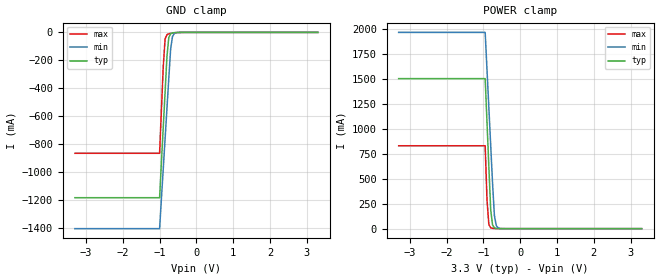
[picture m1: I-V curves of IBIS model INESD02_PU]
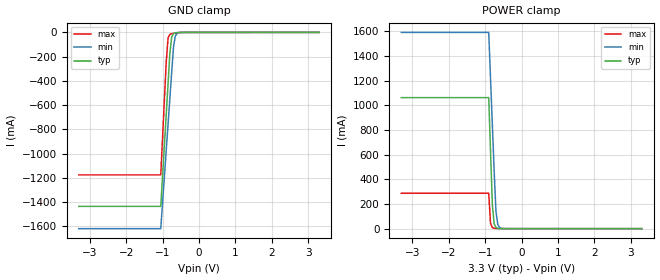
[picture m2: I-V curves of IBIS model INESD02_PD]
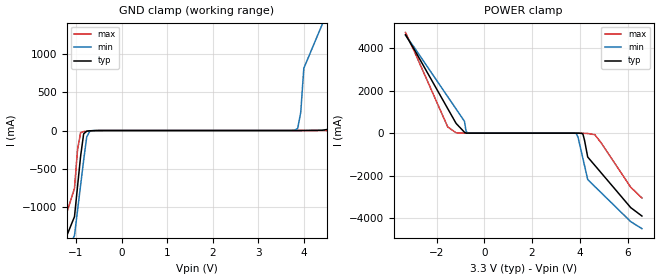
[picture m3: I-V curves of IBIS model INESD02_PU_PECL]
|   This file is an IBIS representation of the   |
|   Integrated Device Technology, Inc.   |
|   ICS844003EI-01   |
|   FEMTOCLOCKS CRYSTAL-TO-LVDS FREQUENCY SYNTHESIZER   |
[IBIS Ver]   4.1
[File name]   844003ei_01_3v3.ibs
[File Rev]   1.0
[Date]   20 Aug 2010
[Source]   Originated at Integrated Device Technology, Inc.
[Disclaimer]
IDT hereby grants the user of this IBIS model a non-exclusive,
nontransferable license to use this IBIS model under the following terms.
Before using this IBIS model, the user should read this license.
If the user does not accept these terms,  the IBIS model should be
returned to IDT within 30 days.
   The user is granted this license only to use the IBIS model and
is not granted rights to sell, load, rent, lease or license the IBIS
model in whole or in part, or in modified form to anyone other than
user. User may modify the IBIS model to suit its specific
applications but rights to derivative works and such modifications
shall belong to IDT.
   This IBIS model is provided on an "AS IS" basis and IDT makes
absolutely no warranty with respect to the information contained
herein. IDT DISCLAIMS AND CUSTOMER WAIVES ALL WARRANTIES, EXPRESS
OR IMPLIED, INCLUDING WARRANTIES OF MERCHANTABILITY OR FITNESS FOR
A PARTICULAR PURPOSE. The entire risk as to quality and performance
is with the Customer. ACCORDINGLY, IN NO EVENT SHALL THE COMPANY BE
LIABLE FOR ANY DAMAGES, WHETHER IN CONTRACT OR TORT,INCLUDING ANY
LOST PROFITS OR OTHER INCIDENTAL, CONSEQUENTIAL, EXEMPLARY, OR
PUNITIVE DAMAGES ARISING OUT OF THE USE OR APPLICATION OF THE IBIS
model provided in this package. Further, IDT reserves the right to
make changes without notice to any product herein to improve
reliability, function, or design. IDT does not convey any license
under patent rights or any other intellectual property rights,
including those of third parties.
   IDT is not obligated to provide maintenance or support
for the licensed IBIS model.
[Copyright]   Copyright 2010 by Integrated Device Technology, Inc.
[Component]   ICS844003EGI-01
[Manufacturer] Integrated Device Technology, Inc.
[Package]
|TSSOP 24 Lead
|   typ   min   max
R_pkg   60.65m   52.4m   68.9m
L_pkg   1.989nH   1.431nH   2.547nH
C_pkg   0.314pF   0.254pF   0.374pF
[Pin] signal_name  model_name   R_pin   L_pin   C_pin
1   DIV_SEL0   INESD02_PU   68.9m   2.547n   0.374p
2   VCO_SEL   INESD02_PU   65.6m   2.323n   0.350p
3   MR   INESD02_PD   62.3m   2.100n   0.326p
4   NC   NC   59.0m   1.877n   0.302p
5   NC   NC   55.7m   1.654n   0.278p
6   NC   NC   52.4m   1.431n   0.254p
7   OE   INESD02_PU_PECL   52.4m   1.431n   0.254p
8   NC   NC   55.7m   1.654n   0.278p
9   FB_DIV   INESD02_PD   59.0m   1.877n   0.302p
10   VDDA   POWER   62.3m   2.100n   0.326p
11   VDD   POWER   65.6m   2.323n   0.350p
12   NC   NC   68.9m   2.547n   0.374p
13   NC   NC   68.9m   2.547n   0.374p
14   GND   GND   65.6m   2.323n   0.350p
15   XTAL_OUT   NC   62.3m   2.100n   0.326p
16   XTAL_IN   NC   59.0m   1.877n   0.302p
17   REF_CLK   INESD02_PD_PECL   55.7m   1.654n   0.278p
18   XTAL_SEL   INESD02_PU   52.4m   1.431n   0.254p
19   nQ1   ONLVDS03_LVDS01_   52.4m   1.431n   0.254p
20   Q1   ONLVDS03_LVDS01_   55.7m   1.654n   0.278p
21   nQ0   ONLVDS03_LVDS01_   59.0m   1.877n   0.302p
22   Q0   ONLVDS03_LVDS01_   62.3m   2.100n   0.326p
23   VDDO   POWER   65.6m   2.323n   0.350p
24   DIV_SEL1   INESD02_PU   68.9m   2.547n   0.374p
[Diff Pin]  inv_pin  vdiff tdelay_typ tdelay_min  tdelay_max
20   19   NA   0  0  0
22   21   NA   0  0  0
| Models and submodels in the file (5): INESD02_PU (Input), INESD02_PD (Input), INESD02_PU_PECL (Input), INESD02_PD_PECL (Input), ONLVDS03_LVDS01_ (Output)
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[Model]   INESD02_PU
Model_type   Input
Polarity   Non-Inverting
Vinl = 0.80V
Vinh = 2.0V
|   typ   min   max
C_comp   2pF   1.5pF   2.5pF
|   typ   min   max
[Voltage range]  3.3V   3.135V   3.465V
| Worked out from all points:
|   GND clamp passes 1 mA (typ) near -0.56 V on its own axis
|   POWER clamp passes 1 mA (typ) near -0.61 V on its own axis
[GND_clamp]
|Voltage   I(typ)   I(min)   I(max)
-3.3V     -1.184A    -1.405A    -865.6mA
-1V       -1.184A    -1.405A    -865.6mA
-900mV    -678.5mA   -975.1mA   -244.1mA
-850mV    -426.2mA   -760.2mA   -46.92mA
-800mV    -174mA     -545.4mA   -16.17mA
-750mV    -37.03mA   -330.8mA   -9.981mA
-700mV    -9.767mA   -120.3mA   -7.122mA
-650mV    -3.616mA   -29.78mA   -4.922mA
-600mV    -1.7mA     -7.594mA   -3.115mA
-400mV    -123.9uA   -126uA     -173.9uA
3.3V      1.866nA    3.949uA    0A
[POWER_clamp]
|Voltage   I(typ)   I(min)   I(max)
-3.3V     1.506A     1.97A      832.1mA
-950mV    1.506A     1.97A      832.1mA
-900mV    1.063A     1.592A     287.2mA
-850mV    620.4mA    1.215A     41.77mA
-800mV    191.5mA    837.4mA    8.692mA
-750mV    37.69mA    460.1mA    3.262mA
-700mV    8.032mA    133.8mA    1.662mA
-650mV    2.005mA    32.58mA    840.1uA
-600mV    607uA      8.009mA    378.6uA
-450mV    33.11uA    139.8uA    23.88uA
3.3V      -71.13uA   -77.46uA   -62.11uA
[Model]   INESD02_PD
Model_type   Input
Polarity   Non-Inverting
Vinl = 0.80V
Vinh = 2.0V
|   typ   min   max
C_comp   2pF   1.5pF   2.5pF
|   typ   min   max
[Voltage range]  3.3V   3.135V   3.465V
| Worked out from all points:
|   GND clamp passes 1 mA (typ) near -0.56 V on its own axis
|   POWER clamp passes 1 mA (typ) near -0.61 V on its own axis
[GND_clamp]
|Voltage   I(typ)   I(min)   I(max)
-3.3V     -1.436A    -1.62A     -1.176A
-1.05V    -1.436A    -1.62A     -1.176A
-900mV    -678.5mA   -975.1mA   -244mA
-850mV    -426.1mA   -760.1mA   -46.85mA
-800mV    -173.9mA   -545.4mA   -16.11mA
-750mV    -36.96mA   -330.7mA   -9.916mA
-700mV    -9.696mA   -120.2mA   -7.056mA
-650mV    -3.545mA   -29.7mA    -4.857mA
-600mV    -1.629mA   -7.52mA    -3.049mA
-400mV    -52.81uA   -52.52uA   -108.7uA
3.3V      71.13uA    77.43uA    62.11uA
[POWER_clamp]
|Voltage   I(typ)   I(min)   I(max)
-3.3V     1.063A     1.593A     287.3mA
-900mV    1.063A     1.593A     287.3mA
-850mV    620.5mA    1.215A     41.84mA
-800mV    191.6mA    837.5mA    8.757mA
-750mV    37.76mA    460.2mA    3.328mA
-700mV    8.104mA    133.8mA    1.728mA
-650mV    2.076mA    32.66mA    905.3uA
-600mV    678.1uA    8.083mA    443.8uA
-450mV    104.2uA    213.3uA    89.09uA
3.3V      -3.041nA   -3.986uA   0A
[Model]   INESD02_PU_PECL
Model_type  Input
Polarity   Non-Inverting
Vinl = 0.8V
Vinh = 2.0V
|   typ   min   max
C_comp   2pF   1.5pF   2.5pF
|   typ   min   max
[Voltage range]  3.3V   3.135V   3.465V
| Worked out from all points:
|   GND clamp passes 1 mA (typ) near -0.59 V on its own axis
|   POWER clamp passes 1 mA (typ) near -0.70 V on its own axis
[GND_clamp]
|Voltage   I(typ)   I(min)   I(max)
-3.3V     -3.894A    -3.674A    -4.294A
-1.3V     -1.521A    -1.7A      -1.261A
-1.031V   -1.125A    -1.372A    -755.3mA
-896.9mV  -335.4mA   -714.7mA   -27.07mA
-695.9mV  -3.401mA   -10.69mA   -6.477mA
3.794V    17.99uA    3.319mA    6.081uA
3.928V    181.1uA    239mA      10.12uA
3.995V    711.6uA    813.7mA    20.78uA
4.8V      40.44mA    1.967A     268.6uA
5.6V      1.139A     3.12A      2.243mA
6.3V      2.525A     4.275A     64.01mA
6.6V      3.219A     4.852A     752.7mA
[POWER_clamp]
|Voltage   I(typ)   I(min)   I(max)
-3.3V     4.617A     4.594A     4.726A
-1.53V    1.149A     1.709A     289.6mA
-1.18V    456.4mA    1.132A     15.33mA
-829.9mV  42.02mA    556.1mA    3.39mA
-762.9mV  4.159mA    91mA       1.422mA
-695.9mV  727.9uA    10.66mA    491.6uA
3.861V    -620.9uA   -26.2mA    -103.4uA
4.129V    -41.91mA   -1.19A     -4.968mA
4.33V     -1.119A    -2.176A    -17.93mA
4.63V     -1.515A    -2.505A    -71.45mA
6.13V     -3.492A    -4.151A    -2.536A
6.6V      -3.888A    -4.48A     -3.041A
